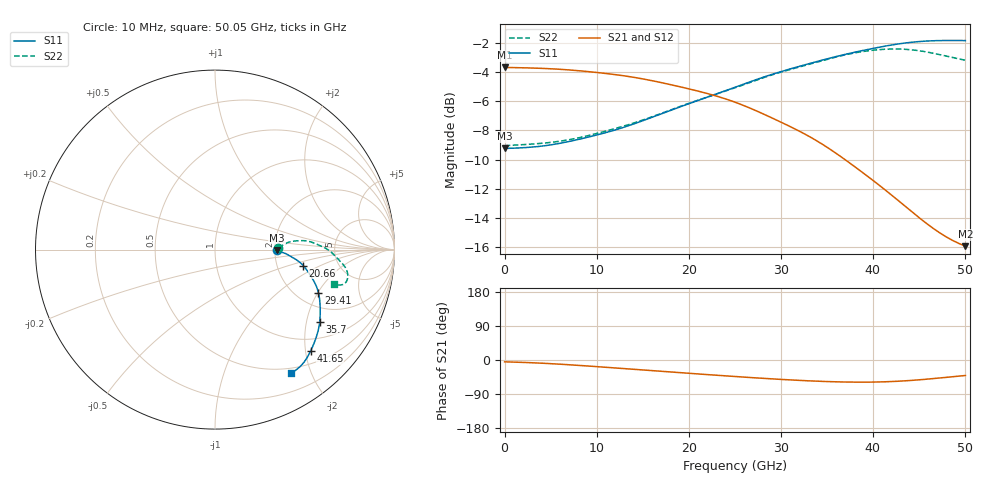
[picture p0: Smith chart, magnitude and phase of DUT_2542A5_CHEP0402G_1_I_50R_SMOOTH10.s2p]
! Touchstone file from project
! Exported from ElectronicsDesktop 2025.1.3
# GHz S MA R 50.000000
! Terminal data exported
! Port[1] = Port1
! Port[2] = Port2
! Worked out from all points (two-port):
!   144 points, 10 MHz to 50.05 GHz, reference 50 ohm
!   highest |S21| = -3.69 dB at 10 MHz (marker M1); lowest = -15.9 dB at 50.05 GHz (marker M2)
!   |S21| within 3 dB of the highest: start of sweep to 27.47 GHz
!   lowest |S11| = -9.2 dB at 10 MHz (marker M3), VSWR 2.06, Z = 103 - j0.433 ohm
!   |S11| at or under -10 dB: nowhere
!   |S22| runs from -9.0 to -2.4 dB; largest |S21 - S12| = 0.0019
!   S11 on the Smith chart (normalised r, x): 10 MHz: 2.06, -0.01; 20.66 GHz: 2.82, -0.67; 29.41 GHz: 2.58, -2.02; 35.7 GHz: 1.49, -2.40; 41.65 GHz: 0.74, -2.10; 50.05 GHz: 0.43, -1.71
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0.01  0.3454 -0.3  0.6537 -4.8  0.6534 -4.8  0.3532 1.6
! Gamma 0 0 0 0
! Port Impedance 50 0 50 0
2.1097  0.3476 -0.6  0.6518 -6.4  0.6512 -6.4  0.3561 1.9
3.85945  0.3514 -1.0  0.6493 -8.2  0.6485 -8.1  0.3594 2.3
5.95915  0.3594 -1.6  0.6444 -10.9  0.6433 -10.8  0.3656 2.8
8.4088  0.3733 -2.2  0.6355 -14.8  0.6344 -14.6  0.3779 3.7
12.6082  0.4048 -3.9  0.6143 -22.0  0.6133 -21.8  0.4091 5.6
16.8076  0.4513 -6.8  0.5821 -29.5  0.5815 -29.3  0.4526 6.1
20.65705  0.4993 -10.2  0.5461 -36.2  0.546 -36.0  0.5007 5.7
23.1067  0.5315 -13.3  0.5207 -40.4  0.5209 -40.2  0.531 4.8
25.2064  0.5617 -16.2  0.495 -43.9  0.4953 -43.7  0.5593 3.5
27.3061  0.5934 -19.2  0.4652 -47.2  0.4656 -47.0  0.5907 1.9
29.4058  0.624 -22.6  0.434 -50.3  0.4345 -50.2  0.6215 0.4
31.5055  0.6525 -26.4  0.4033 -53.2  0.4038 -53.0  0.6495 -1.4
33.6052  0.6805 -30.5  0.3717 -55.6  0.3719 -55.5  0.6772 -3.6
35.7049  0.7083 -34.5  0.3375 -57.4  0.3375 -57.3  0.7057 -5.7
38.85445  0.7463 -40.9  0.2864 -58.5  0.2858 -58.4  0.7403 -8.6
41.65405  0.7763 -46.6  0.2447 -57.2  0.2439 -57.0  0.7551 -11.6
42.004  0.7797 -47.3  0.2398 -56.9  0.2389 -56.7  0.7557 -12.0
43.75375  0.7941 -50.3  0.216 -54.6  0.2151 -54.3  0.7531 -13.8
45.5035  0.8034 -52.9  0.1949 -51.4  0.194 -51.0  0.7415 -15.1
47.95315  0.8083 -56.0  0.1724 -45.8  0.1715 -45.5  0.715 -16.0
50.05285  0.8075 -58.2  0.1601 -40.9  0.1594 -40.5  0.6915 -16.2
